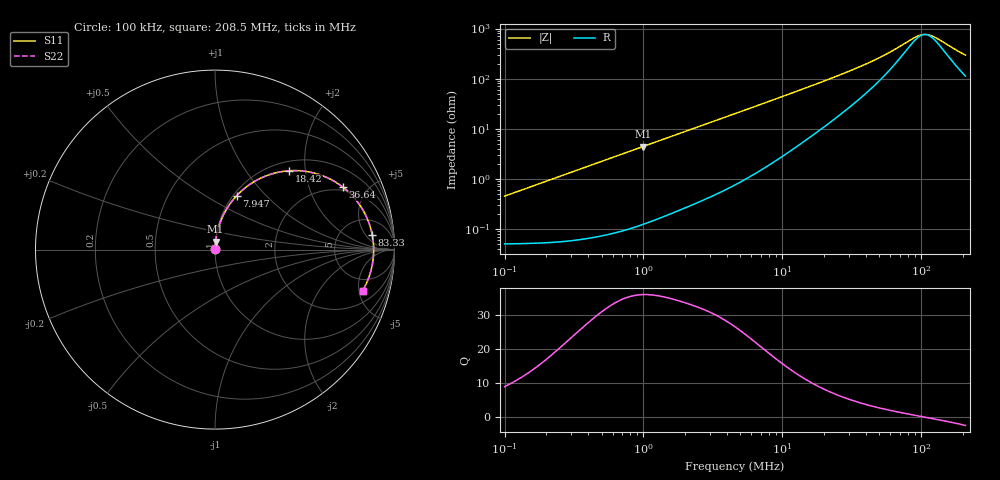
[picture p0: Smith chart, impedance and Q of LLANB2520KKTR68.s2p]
! LLANB2520KKTR68  S-PARAMETER MODEL  ( General Type )
! Model Generated by TAIYO YUDEN Corporation (http://www.ty-top.com)
! Version 3.0
! TAIYO YUDEN Control No. 20210629
! Copyright(c) 2013 TAIYO YUDEN CO.,LTD. All Rights Reserved.
! Product Description (link to TY-COMPAS)
! https://ds.yuden.co.jp/TYCOMPAS/or/detail?pn=LLANB2520KKTR68M&u=M
! Products Name : Inductors
! Characteristics :
!  Inductance : 0.68 uH , SRF(min) : -Hz , DC Resistance(max) : 0.059 Ohm
!  Rated Current : Saturation :3700 mA , Temp Rise : 2900 mA (40 degC)
!  Case Size : 2.5 x 2.0 / 0.098 x 0.079 [mm/inch] , Thickness : 1 / 0.039 [mm/inch]
!  (Conditions: Temperature = 25 degC , DC Bias Current/Voltage = 0A / 0V)
! External Node Assignments :
!  1  o---GGG---o  2
! GND o---------o GND
! Frequency Range : 0.1MHz  -  208.503118MHz  [ 402 STEP ]
# MHz S RI R 50
! Freq[MHz].  S11 Real  S11 Imag  S21 Real  S21 Imag  S12 Real  S12 Imag  S22 Real  S22 Imag
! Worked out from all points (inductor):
!   401 points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, 100 kHz to 208.5 MHz, reference 50 ohm
!   read as one part in series: L = 709 nH near 103.9 kHz
!   highest Q = 36 at 990.2 kHz (marker M1), where L = 704 nH
!   self-resonance near 106.5 MHz
!   S11 on the Smith chart (normalised r, x): 100 kHz: 1.00, +0.01; 7.947 MHz: 1.04, +0.69; 18.42 MHz: 1.18, +1.63; 36.64 MHz: 1.82, +3.41; 83.33 MHz: 10, +7; 208.5 MHz: 3.24, -5.46
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0.1  0.000517 0.00445  0.9995 -0.00445  0.9995 -0.00445  0.000517 0.00445
0.359709  0.00087 0.016  0.9991 -0.016  0.9991 -0.016  0.00087 0.016
0.990225  0.00313 0.0436  0.9969 -0.0436  0.9969 -0.0436  0.00313 0.0436
1.293906  0.00484 0.0567  0.9952 -0.0567  0.9952 -0.0567  0.00484 0.0567
2.574085  0.0159 0.1105  0.9841 -0.1105  0.9841 -0.1105  0.0159 0.1105
4.654297  0.0463 0.192  0.9537 -0.192  0.9537 -0.192  0.0463 0.192
7.946794  0.1199 0.2994  0.8801 -0.2994  0.8801 -0.2994  0.1199 0.2994
11.42483  0.2167 0.3778  0.7833 -0.3778  0.7833 -0.3778  0.2167 0.3778
16.42508  0.3592 0.4323  0.6408 -0.4323  0.6408 -0.4323  0.3592 0.4323
18.4202  0.4114 0.4392  0.5886 -0.4392  0.5886 -0.4392  0.4114 0.4392
25.48922  0.5637 0.4234  0.4363 -0.4234  0.4363 -0.4234  0.5637 0.4234
36.64498  0.7122 0.3484  0.2878 -0.3484  0.2878 -0.3484  0.7122 0.3484
46.97704  0.7872 0.2746  0.2128 -0.2746  0.2128 -0.2746  0.7872 0.2746
59.08252  0.8357 0.1993  0.1643 -0.1993  0.1643 -0.1993  0.8357 0.1993
83.33339  0.8757 0.0831  0.1243 -0.0831  0.1243 -0.0831  0.8757 0.0831
91.68704  0.8808 0.0508  0.1192 -0.0508  0.1192 -0.0508  0.8808 0.0508
98.96898  0.8831 0.0249  0.1169 -0.0249  0.1169 -0.0249  0.8831 0.0249
106.8293  0.884 -0.000907  0.116 0.000907  0.116 0.000907  0.884 -0.000907
115.3138  0.8833 -0.0268  0.1167 0.0268  0.1167 0.0268  0.8833 -0.0268
129.3207  0.8794 -0.0657  0.1206 0.0657  0.1206 0.0657  0.8794 -0.0657
178.9494  0.8486 -0.1765  0.1514 0.1765  0.1514 0.1765  0.8486 -0.1765
208.5031  0.8224 -0.2285  0.1776 0.2285  0.1776 0.2285  0.8224 -0.2285
